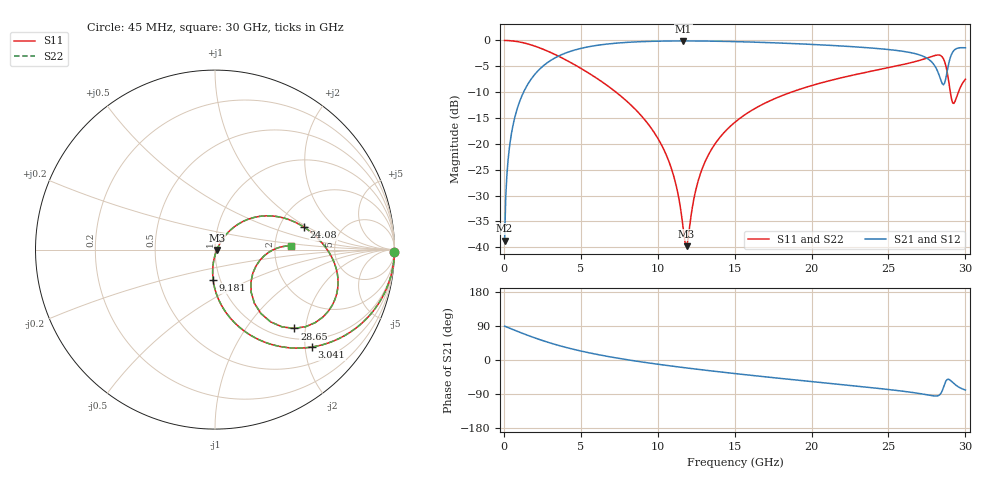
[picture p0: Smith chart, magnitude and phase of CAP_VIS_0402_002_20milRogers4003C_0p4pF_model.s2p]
! S-parameter model data by Modelithics Inc.  support@modelithics.com  813-866-6335  Tampa FL USA
! S-Parameter data specifications:
! Substrate: 20-mil Rogers 4003C, substrate thickness, H=0.508mm, Dielectric constant, Er=3.75
! PCB Mounting Pad Footprint: Pad width, PadW=0.50mm , Pad length, PadL=0.50mm , Pad gap, PadG (edge-to-edge)=0.40mm , Reference planes=1.4mm apart
! Created Wed Nov 18 12:41:26 2015
# hz S ma R 50
! 2 Port Network Data from SP1.SP block
! freq  magS11  angS11  magS21  angS21  magS12  angS12  magS22  angS22
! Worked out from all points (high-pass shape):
!   401 points, 45 MHz to 30 GHz, reference 50 ohm
!   highest |S21| = -0.09 dB at 11.65 GHz (marker M1); lowest = -38.7 dB at 45 MHz (marker M2)
!   |S21| within 3 dB of the highest: 3.503 GHz to 27.28 GHz (23.77 GHz wide, 154 % of centre); 29.05 GHz to end of sweep
!   lowest |S11| = -39.8 dB at 11.88 GHz (marker M3), VSWR 1.02, Z = 51 - j0.259 ohm
!   |S11| at or under -10 dB: 7.287 GHz to 18.68 GHz (11.4 GHz wide, 87.8 % of centre); 29.02 GHz to 29.54 GHz (522.1 MHz wide, 1.78 % of centre)
!   |S22| runs from -39.8 to 0.0 dB; largest |S21 - S12| = 0
!   S11 on the Smith chart (normalised r, x): 45 MHz: open; 3.041 GHz: 0.82, -2.14; 9.181 GHz: 0.93, -0.32; 24.08 GHz: 2.74, +0.93; 28.65 GHz: 1.21, -1.74; 30 GHz: 2.45, +0.12
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4.5e7  0.9999 -0.7  0.01161 89.3  0.01161 89.3  0.9999 -0.7
3.4455e8  0.996 -5.7  0.08864 84.3  0.08864 84.3  0.996 -5.7
8.687625e8  0.9754 -14.2  0.2198 75.7  0.2198 75.7  0.9754 -14.2
1.767412e9  0.9057 -28.1  0.4221 61.8  0.4221 61.8  0.9057 -28.1
3.0405e9  0.765 -45.2  0.6407 44.5  0.6407 44.5  0.765 -45.2
5.062462e9  0.5309 -66.3  0.8419 23.1  0.8419 23.1  0.5309 -66.3
9.181275e9  0.1691 -93.5  0.9767 -6.5  0.9767 -6.5  0.1691 -93.5
1.007992e10  0.1083 -96.7  0.9847 -11.6  0.9847 -11.6  0.1083 -96.7
1.105346e10  0.04788 -95.1  0.9888 -16.8  0.9888 -16.8  0.04788 -95.1
1.165256e10  0.01537 -69.0  0.9895 -19.9  0.9895 -19.9  0.01537 -69.0
1.187722e10  0.01024 -14.3  0.9895 -21.0  0.9895 -21.0  0.01024 -14.3
1.247632e10  0.03592 49.1  0.9885 -24.0  0.9885 -24.0  0.03592 49.1
1.300054e10  0.06319 53.7  0.9869 -26.5  0.9869 -26.5  0.06319 53.7
1.50225e10  0.162 50.0  0.9747 -35.8  0.9747 -35.8  0.162 50.0
2.003996e10  0.3674 30.7  0.9154 -57.1  0.9154 -57.1  0.3674 30.7
2.408389e10  0.5114 14.2  0.8406 -73.8  0.8406 -73.8  0.5114 14.2
2.505742e10  0.5479 9.7  0.8153 -78.1  0.8153 -78.1  0.5479 9.7
2.797804e10  0.7129 -16.0  0.5769 -95.0  0.5769 -95.0  0.7129 -16.0
2.865202e10  0.6231 -44.8  0.3881 -63.1  0.3881 -63.1  0.6231 -44.8
2.895158e10  0.3706 -53.7  0.6285 -51.6  0.6285 -51.6  0.3706 -53.7
2.925112e10  0.246 -21.8  0.7986 -62.2  0.7986 -62.2  0.246 -21.8
3e10  0.4215 2.7  0.8483 -79.2  0.8483 -79.2  0.4215 2.7
